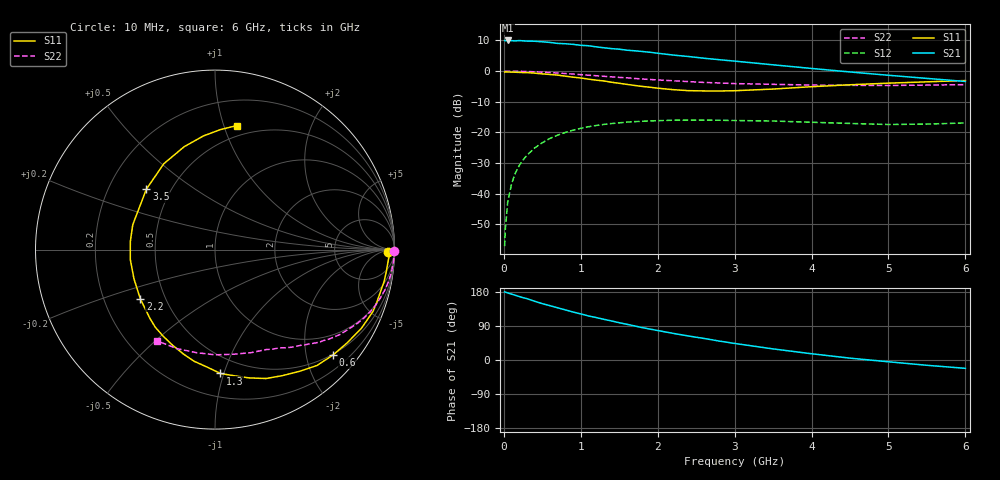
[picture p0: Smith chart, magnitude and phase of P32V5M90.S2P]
! SIEMENS Small Signal Semiconductors
! BFP181
! Si NPN RF Bipolar Junction Transistor in SOT143
! VCE = 2.5 V  IC = 0.9 mA
! Common Emitter S-Parameters:  March  1996
# GHz  S  MA  R  50
!  f  S11  S21  S12  S22
! GHz  MAG  ANG  MAG  ANG  MAG  ANG  MAG  ANG
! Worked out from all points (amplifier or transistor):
!   36 points, 10 MHz to 6 GHz, reference 50 ohm
!   highest |S21| = 10.0 dB at 50 MHz (marker M1)
!   |S21| within 3 dB of that: start of sweep to 1.546 GHz
!   unconditionally stable (mu >= 1): 3.212 GHz to end of sweep
!   at 250 MHz: K = 0.08, MSG = 19.4 dB, |S12| = -29.0 dB
!   at 1.4 GHz: K = 0.49, MSG = 12.2 dB, |S12| = -17.1 dB
!   at 6 GHz: K = 1.32, MAG = 3.4 dB, |S12| = -16.9 dB
!   S11 on the Smith chart (normalised r, x): 10 MHz: 49, -19; 600 MHz: 0.48, -2.54; 1.3 GHz: 0.37, -0.97; 2.2 GHz: 0.36, -0.26; 3.5 GHz: 0.37, +0.33; 6 GHz: 0.41, +1.11
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0.01  0.9654 -0.8  3.155 179.7  0.0014 80.0  0.9978 -0.3
0.02  0.9733 -1.7  3.129 179.3  0.0027 90.9  0.9916 -0.6
0.05  0.9675 -3.4  3.159 176.9  0.0073 90.5  0.9964 -1.7
0.1  0.9624 -7.2  3.132 173.9  0.0144 85.1  0.998 -3.3
0.2  0.9515 -14.3  3.146 167.5  0.0289 80.6  0.9919 -6.7
0.4  0.9263 -28.2  3.068 155.0  0.0558 71.2  0.9744 -13.1
0.5  0.9009 -35.3  3.004 148.7  0.068 66.7  0.9604 -16.2
0.6  0.8815 -41.8  2.932 143.3  0.08 62.0  0.9466 -19.2
0.9  0.7966 -61.8  2.728 126.6  0.109 50.1  0.8949 -27.2
1.1  0.7393 -75.2  2.588 116.3  0.1239 43.1  0.8576 -31.9
1.3  0.6909 -87.5  2.401 107.4  0.1352 36.3  0.823 -36.3
1.5  0.6329 -100.6  2.276 98.4  0.1434 31.0  0.7895 -39.9
1.8  0.5627 -120.7  2.085 85.4  0.1521 23.9  0.7439 -44.9
2.2  0.4982 -146.7  1.827 70.3  0.1583 15.5  0.6961 -51.2
2.4  0.4799 -160.2  1.729 63.4  0.159 12.0  0.6748 -54.2
2.8  0.4739 174.6  1.534 50.0  0.1581 6.5  0.6409 -59.9
3  0.4787 163.2  1.455 43.7  0.1565 3.8  0.6258 -62.8
3.5  0.5095 138.6  1.266 29.3  0.1536 -0.6  0.6086 -70.6
4  0.557 120.8  1.105 16.5  0.1466 -3.7  0.5923 -79.7
4.5  0.5984 106.7  0.968 4.9  0.1402 -5.3  0.5864 -89.9
5.5  0.6685 87.6  0.76 -14.0  0.1369 -1.7  0.5913 -111.2
6  0.7019 80.0  0.678 -22.0  0.1429 -0.3  0.6018 -122.3
